PROGRAM MAIN
VAR
	AODB			: ARRAY[0..49] OF ST_IEC870_5_101AODBEntry;(* Application object data base (data points)*)
	hServer			: T_HSERVER;(* Server connection handle *)
	fbServer		: FB_IEC870_5_104SlaveGrp;(* IEC 60870-5-104 controlled station function block instance *)
	aConnections	: ARRAY[0..1] OF ST_IEC870_5_104ServerConnection; (* Two master connections *)

	nCAA			: UDINT := 7;(* Common ASDU address of local (slave) station *)

	inputs AT%I*	: ARRAY[0..2999] OF BYTE;
	outputs AT%Q*	: ARRAY[0..2999] OF BYTE;
	memory AT%M*	: ST_MemoryData;
	data 			: ARRAY[0..2999] OF BYTE;

	bEnable			: BOOL := TRUE;(* Enables/disables communication/data exchange *)
	bBlock			: BOOL;(* Quality flags sample: Rising edge sets BL quality flag to 1 *)
	bUnblock		: BOOL;(* Quality flags sample: Rising edge resets BL quality flag to 0 *)
	bIsBlocked		: BOOL;(* Quality flags sample: BL quality flag status information (TRUE => BL == 1, FALSE => BL == 0) *)
	bSendSpont		: BOOL;(* Sample: TRUE => simulate/modify plc process data (send spontanous data) *)

	fbTimer			: TON := ( PT := T#10S );
	bInit			: BOOL := TRUE;
	nInitErr		: UDINT;
END_VAR

IF bInit THEN
	bInit := FALSE;

	F_CreateServerHnd( '',(* TwinCAT network adress of TCP/IP server, Default = empty string *)
						'127.0.0.1',(* Local (server) address. String containing an (Ipv4) Internet Protocol dotted address. *)
						2404,(* Local (server) Internet Protocol (IP) port. Default = 2404 *)
						nMode := LISTEN_MODE_CLOSEALL OR CONNECT_MODE_ENABLEDBG,(* Close all previous (old) connections and enable debug messages *)
						bEnable, 
						hServer );

	(* Configure protocol parameter *)
	fbServer.protPara.t0				:= T#30S;(* MASTER only: Connection establishment, Default = 30s *)
	fbServer.protPara.t1 				:= T#15S;(* Response Timeout (STARTDTAct, STOPDTAct, TESTFRAct only, Default = 15s ) *)
	fbServer.protPara.t2 				:= T#10S;(* Send ACK in case of no data frames, Default = 10s *)
	fbServer.protPara.t3 				:= T#20S;(* Time for sending test frames, Default = 20s *)
	fbServer.protPara.iK 				:= 12;(* Max. difference RSN to send ACK, Default = 12 *)
	fbServer.protPara.iW 				:= 8;(* Latest ACK after receiving I-frames, Default = 8 *)
	fbServer.protPara.bThrottleMode 	:= TRUE;(* If set reduces the number of polling socket read requests *)
	fbServer.protPara.bPackFrames 		:= TRUE;(* Binds more than one APDU frame to one big TCP/IP frame *)

	(* Configure system parameter *)
	fbServer.sysPara.asduAddr 			:= nCAA;(* Own common ASDU address *)
	fbServer.sysPara.asduFmt.eCOTSize 		:= eIEC870_COT_TwoOctets;(* Cause of transfer octet size *)
	fbServer.sysPara.asduFmt.eAsduAddrSize 	:= eIEC870_AsduAddr_TwoOctets;(* Common ASDU address octet size *)
	fbServer.sysPara.asduFmt.eObjAddrSize 	:= eIEC870_ObjAddr_ThreeOctets;(* Object address octet size *)

	fbServer.sysPara.bUsePCTime 		:= TRUE;(* Initialize substation clock with PC time *)
	fbServer.sysPara.bSyncTime 			:= TRUE;(* Clock synchronisation command enabled *)
	fbServer.sysPara.bSyncPCTime 		:= FALSE;(* Synchronisation of PC time disabled *)
	fbServer.sysPara.bTimeCOT3 			:= FALSE;(* Transmission of C_CS_NA_1 with COT = spontanous disabled *)

	fbServer.sysPara.bEndOfInit 		:= TRUE;(* Send end of initialization *)

	fbServer.sysPara.bPerCyclic			:= FALSE;(* Periodic, cyclic data transfer disabled *)
	fbServer.sysPara.tPerCyclicBase		:= T#5S;(* Periodic, cyclic data transfer base time *)

	fbServer.sysPara.bBackScan			:= FALSE;(* Background scan disabled *)
	fbServer.sysPara.tBackScanCycle		:= T#30S;(* Background scan cycle time *)

	fbServer.sysPara.bPerFRZ			:= TRUE;(* Periodic freeze/reset of integrated totals enabled *)
	fbServer.sysPara.tPerFRZCycle		:= T#15S;(* Perdiodic freeze/reset of integrate totals cycle time *)

	
	fbServer.sysPara.dbgMode 			:= IEC870_DEBUGMODE_DEVSTATE OR IEC870_DEBUGMODE_LINKERROR(* OR IEC870_DEBUGMODE_ASDU OR IEC870_DEBUGMODE_LINKLAYER *); 



	(* Configure your IEC data points here: *)

	(* Monitored Single Points *)
	nInitErr := F_iecInitAOEntry( M_SP_NA_1, 100, IEC870_GRP_INROGEN, 0, MAP_AREA_MEMORY, ADR( memory.eSPI_100_msg ) - ADR( memory ), 0, AODB[0] );
	nInitErr := F_iecInitAOEntry( M_SP_NA_1, 101, IEC870_GRP_INROGEN, 0, MAP_AREA_MEMORY, ADR( memory.eSPI_101_msg ) - ADR( memory ), 0, AODB[1] );
	nInitErr := F_iecInitAOEntry( M_SP_TB_1, 102, IEC870_GRP_INROGEN, 0, MAP_AREA_MEMORY, ADR( memory.eSPI_102_msg ) - ADR( memory ), 0, AODB[2] );
	(* Double Points*)
	nInitErr := F_iecInitAOEntry( M_DP_NA_1, 200, IEC870_GRP_INROGEN, 0, MAP_AREA_MEMORY, ADR( memory.eDPI_200_msg ) - ADR( memory ), 0, AODB[3] );
	nInitErr := F_iecInitAOEntry( M_DP_NA_1, 201, IEC870_GRP_INROGEN, 0, MAP_AREA_MEMORY, ADR( memory.eDPI_201_msg ) - ADR( memory ), 0, AODB[4] );
	nInitErr := F_iecInitAOEntry( M_DP_TB_1, 202, IEC870_GRP_INROGEN, 0, MAP_AREA_MEMORY, ADR( memory.eDPI_202_msg ) - ADR( memory ), 0, AODB[5] );
	(* Regulating step value *)
	nInitErr := F_iecInitAOEntry( M_ST_NA_1, 300, IEC870_GRP_INROGEN, 0, MAP_AREA_MEMORY, ADR( memory.nVTI_300_msg ) - ADR( memory ), 0, AODB[6] );
	nInitErr := F_iecInitAOEntry( M_ST_NA_1, 301, IEC870_GRP_INROGEN, 0, MAP_AREA_MEMORY, ADR( memory.nVTI_301_msg ) - ADR( memory ), 0, AODB[7] );
	nInitErr := F_iecInitAOEntry( M_ST_TB_1, 302, IEC870_GRP_INROGEN, 0, MAP_AREA_MEMORY, ADR( memory.nVTI_302_msg ) - ADR( memory ), 0, AODB[8] );
	(* 32 bit string*)
	nInitErr := F_iecInitAOEntry( M_BO_NA_1, 400, IEC870_GRP_INROGEN, 0, MAP_AREA_MEMORY, ADR( memory.nBSI_400_msg ) - ADR( memory ), 0, AODB[9] );
	nInitErr := F_iecInitAOEntry( M_BO_NA_1, 401, IEC870_GRP_INROGEN, 0, MAP_AREA_MEMORY, ADR( memory.nBSI_401_msg ) - ADR( memory ), 0, AODB[10] );
	nInitErr := F_iecInitAOEntry( M_BO_TB_1, 402, IEC870_GRP_INROGEN, 0, MAP_AREA_MEMORY, ADR( memory.nBSI_402_msg ) - ADR( memory ), 0, AODB[11] );
	(* Measured value, normalized value *)
	nInitErr := F_iecInitAOEntry( M_ME_NA_1, 500, IEC870_GRP_INROGEN, 0, MAP_AREA_MEMORY, ADR( memory.nNVA_500_msg ) - ADR( memory ), 0, AODB[12] );
	nInitErr := F_iecInitAOEntry( M_ME_NA_1, 501, IEC870_GRP_INROGEN, 0, MAP_AREA_MEMORY, ADR( memory.nNVA_501_msg ) - ADR( memory ), 0, AODB[13] );
	nInitErr := F_iecInitAOEntry( M_ME_TD_1, 502, IEC870_GRP_INROGEN, 0, MAP_AREA_MEMORY, ADR( memory.nNVA_502_msg ) - ADR( memory ), 0, AODB[14] );
	(* Mesured value, scaled value *)
	nInitErr := F_iecInitAOEntry( M_ME_NB_1, 600, IEC870_GRP_INROGEN, 0, MAP_AREA_MEMORY, ADR( memory.nSVA_600_msg ) - ADR( memory ), 0, AODB[15] );
	nInitErr := F_iecInitAOEntry( M_ME_NB_1, 601, IEC870_GRP_INROGEN, 0, MAP_AREA_MEMORY, ADR( memory.nSVA_601_msg ) - ADR( memory ), 0, AODB[16] );
	nInitErr := F_iecInitAOEntry( M_ME_TE_1, 602, IEC870_GRP_INROGEN, 0, MAP_AREA_MEMORY, ADR( memory.nSVA_602_msg ) - ADR( memory ), 0, AODB[17] );
	(* Measured value , short floating point value *)
	nInitErr := F_iecInitAOEntry( M_ME_NC_1, 700, IEC870_GRP_INROGEN, 0, MAP_AREA_MEMORY, ADR( memory.fR32_700_msg ) - ADR( memory ), 0, AODB[18] );
	nInitErr := F_iecInitAOEntry( M_ME_NC_1, 701, IEC870_GRP_INROGEN, 0, MAP_AREA_MEMORY, ADR( memory.fR32_701_msg ) - ADR( memory ), 0, AODB[19] );
	nInitErr := F_iecInitAOEntry( M_ME_TF_1, 702, IEC870_GRP_INROGEN, 0, MAP_AREA_MEMORY, ADR( memory.fR32_702_msg ) - ADR( memory ), 0, AODB[20] );

	(* Integrated totals *)
	(* We configure the Mode A: local freeze and spontanous data transfer *)
	nInitErr := F_iecInitAOEntry( M_IT_NA_1, 800, IEC870_GRP_REQCOGEN OR IEC870_GRP_LOCFREEZE, 0, MAP_AREA_MEMORY, ADR( memory.nBCR_800_msg ) - ADR( memory ), 0, AODB[21] );
	nInitErr := F_iecInitAOEntry( M_IT_NA_1, 801, IEC870_GRP_REQCOGEN OR IEC870_GRP_LOCFREEZE, 0, MAP_AREA_MEMORY, ADR( memory.nBCR_801_msg ) - ADR( memory ), 0, AODB[22] );
	nInitErr := F_iecInitAOEntry( M_IT_TB_1, 802, IEC870_GRP_REQCOGEN OR IEC870_GRP_LOCFREEZE, 0, MAP_AREA_MEMORY, ADR( memory.nBCR_802_msg ) - ADR( memory ), 0, AODB[23] );

	(* Controlled Single commands *)
	nInitErr := F_iecInitAOEntry( C_SC_NA_1, 10, 0, 0, MAP_AREA_MEMORY, ADR( memory.eSCS_10_cmd ) - ADR( memory ), 0, AODB[24] );
	nInitErr := F_iecInitAOEntry( C_SC_NA_1, 11, 0, 0, MAP_AREA_MEMORY, ADR( memory.eSCS_11_cmd ) - ADR( memory ), 0, AODB[25] );
	nInitErr := F_iecInitAOEntry( C_SC_TA_1, 12, 0, 0, MAP_AREA_MEMORY, ADR( memory.eSCS_12_cmd ) - ADR( memory ), 0, AODB[26] );
	(* Double commands *)
	nInitErr := F_iecInitAOEntry( C_DC_NA_1, 20, 0, 0, MAP_AREA_MEMORY, ADR( memory.eDCS_20_cmd ) - ADR( memory ), 0, AODB[27] );
	nInitErr := F_iecInitAOEntry( C_DC_NA_1, 21, 0, 0, MAP_AREA_MEMORY, ADR( memory.eDCS_21_cmd ) - ADR( memory ), 0, AODB[28] );
	nInitErr := F_iecInitAOEntry( C_DC_TA_1, 22, 0, 0, MAP_AREA_MEMORY, ADR( memory.eDCS_22_cmd ) - ADR( memory ), 0, AODB[29] );
	(* Regulating step commands *)
	nInitErr := F_iecInitAOEntry( C_RC_NA_1, 30, 0, 0, MAP_AREA_MEMORY, ADR( memory.nVTI_30_cmd ) - ADR( memory ), 0, AODB[30] );
	nInitErr := F_iecInitAOEntry( C_RC_NA_1, 31, 0, 0, MAP_AREA_MEMORY, ADR( memory.nVTI_31_cmd ) - ADR( memory ), 0, AODB[31] );
	nInitErr := F_iecInitAOEntry( C_RC_TA_1, 32, 0, 0, MAP_AREA_MEMORY, ADR( memory.nVTI_32_cmd ) - ADR( memory ), 0, AODB[32] );
	(* 32 bit string commands *)
	nInitErr := F_iecInitAOEntry( C_BO_NA_1, 40, 0, 0, MAP_AREA_MEMORY, ADR( memory.nBSI_40_cmd ) - ADR( memory ), 0, AODB[33] );
	nInitErr := F_iecInitAOEntry( C_BO_NA_1, 41, 0, 0, MAP_AREA_MEMORY, ADR( memory.nBSI_41_cmd ) - ADR( memory ), 0, AODB[34] );
	nInitErr := F_iecInitAOEntry( C_BO_TA_1, 42, 0, 0, MAP_AREA_MEMORY, ADR( memory.nBSI_42_cmd ) - ADR( memory ), 0, AODB[35] );
	(* Set point,  normalized values*)
	nInitErr := F_iecInitAOEntry( C_SE_NA_1, 50, 0, 0, MAP_AREA_MEMORY, ADR( memory.nNVA_50_cmd ) - ADR( memory ), 0, AODB[36] );
	nInitErr := F_iecInitAOEntry( C_SE_NA_1, 51, 0, 0, MAP_AREA_MEMORY, ADR( memory.nNVA_51_cmd ) - ADR( memory ), 0, AODB[37] );
	nInitErr := F_iecInitAOEntry( C_SE_TA_1, 52, 0, 0, MAP_AREA_MEMORY, ADR( memory.nNVA_52_cmd ) - ADR( memory ), 0, AODB[38] );
	(* Set point,  scaled valuess *)
	nInitErr := F_iecInitAOEntry( C_SE_NB_1, 60, 0, 0, MAP_AREA_MEMORY, ADR( memory.nSVA_60_cmd ) - ADR( memory ), 0, AODB[39] );
	nInitErr := F_iecInitAOEntry( C_SE_NB_1, 61, 0, 0, MAP_AREA_MEMORY, ADR( memory.nSVA_61_cmd ) - ADR( memory ), 0, AODB[40] );
	nInitErr := F_iecInitAOEntry( C_SE_TB_1, 62, 0, 0, MAP_AREA_MEMORY, ADR( memory.nSVA_62_cmd ) - ADR( memory ), 0, AODB[41] );
	(* Set point,  short floating point values *)
	nInitErr := F_iecInitAOEntry( C_SE_NC_1, 70, 0, 0, MAP_AREA_MEMORY, ADR( memory.fR32_70_cmd ) - ADR( memory ), 0, AODB[42] );
	nInitErr := F_iecInitAOEntry( C_SE_NC_1, 71, 0, 0, MAP_AREA_MEMORY, ADR( memory.fR32_71_cmd ) - ADR( memory ), 0, AODB[43] );
	nInitErr := F_iecInitAOEntry( C_SE_TC_1, 72, 0, 0, MAP_AREA_MEMORY, ADR( memory.fR32_72_cmd ) - ADR( memory ), 0, AODB[44] );

ELSE
	(* Execute IEC slave function block *)
	fbServer( 	pInputs 		:= ADR( inputs ),
				cbInputs 		:= SIZEOF( inputs ),
				pOutputs 		:= ADR( outputs ),
				cbOutputs 		:= SIZEOF( outputs ),
				pMemory 		:= ADR( memory ),
				cbMemory 		:= SIZEOF( memory ),
				pData 			:= ADR( data ),
				cbData 			:= SIZEOF( data ),
				pAOEntries 		:= ADR( AODB ),
				cbAOEntries 	:= SIZEOF( AODB ),
				pConnections 	:= ADR( aConnections ),
				cbConnections 	:= SIZEOF( aConnections ),
				hServer 		:= hServer,
				bEnable 		:= bEnable );

	(* Check for device errors *)
	REPEAT
		fbServer.system.device.errors.RemoveError();
		IF fbServer.system.device.errors.bOk  THEN
			ADSLOGSTR( 	ADSLOG_MSGTYPE_ERROR OR ADSLOG_MSGTYPE_LOG, 'IEC60870-5-104 slave error: 0x%s',
						DWORD_TO_HEXSTR( fbServer.system.device.errors.getError.nErrId, 8, FALSE) );
		END_IF
	UNTIL NOT fbServer.system.device.errors.bOk
	END_REPEAT

	(* Set block quality flag *)					
	IF bBlock THEN
		bBlock := FALSE;
		F_iecSetAOQuality( IECQ_BL_ON, AODB[0], fbServer.system.device );
	END_IF

	(* Clear block quality flag *)
	IF bUnblock THEN
		bUnblock := FALSE;
		F_iecSetAOQuality( IECQ_BL_OFF, AODB[0], fbServer.system.device );
	END_IF

	(* Check if block quality flag is set *)
	bIsBlocked := SEL( ( F_iecGetAOQuality( AODB[0], fbServer.system.device ) AND IECQ_BL_ON )  = IECQ_BL_ON, FALSE, TRUE );

END_IF

(* Simulate/modify plc process data *)
fbTimer( IN := bSendSpont );
IF fbTimer.Q THEN
	fbTimer( IN := FALSE );
	fbTimer( IN := bSendSpont );

	memory.eSPI_100_msg := SEL( memory.eSPI_100_msg = eIEC870_SPI_OFF, eIEC870_SPI_OFF, eIEC870_SPI_ON );
	memory.eSPI_101_msg := SEL( memory.eSPI_101_msg = eIEC870_SPI_OFF, eIEC870_SPI_OFF, eIEC870_SPI_ON );
	memory.eSPI_102_msg := SEL( memory.eSPI_102_msg = eIEC870_SPI_OFF, eIEC870_SPI_OFF, eIEC870_SPI_ON );

	memory.eDPI_200_msg := SEL( memory.eDPI_200_msg = eIEC870_DPI_OFF, eIEC870_DPI_OFF, eIEC870_DPI_ON );
	memory.eDPI_201_msg := SEL( memory.eDPI_201_msg = eIEC870_DPI_OFF, eIEC870_DPI_OFF, eIEC870_DPI_ON );
	memory.eDPI_202_msg := SEL( memory.eDPI_202_msg = eIEC870_DPI_OFF, eIEC870_DPI_OFF, eIEC870_DPI_ON );
	
	F_iecIncVTI( memory.nVTI_300_msg );
	F_iecDecVTI( memory.nVTI_301_msg );
	F_iecIncVTI( memory.nVTI_302_msg );

	memory.nBSI_400_msg := SEL( memory.nBSI_400_msg = 0, ROL( memory.nBSI_400_msg, 1 ), 16#11111111 );
	memory.nBSI_401_msg := SEL( memory.nBSI_401_msg = 0, ROR( memory.nBSI_401_msg, 1 ), 16#22222222 );
	memory.nBSI_402_msg := SEL( memory.nBSI_402_msg = 0, ROL( memory.nBSI_402_msg, 1 ), 16#33333333 );

	memory.nNVA_500_msg := memory.nNVA_500_msg + 1;
	memory.nNVA_501_msg := memory.nNVA_501_msg - 1;
	memory.nNVA_502_msg := memory.nNVA_502_msg + 2;

	memory.nSVA_600_msg := memory.nSVA_600_msg + 1;
	memory.nSVA_601_msg := memory.nSVA_601_msg - 1;
	memory.nSVA_602_msg := memory.nSVA_602_msg + 2;

	memory.fR32_700_msg	:= memory.fR32_700_msg + 0.1;
	memory.fR32_701_msg	:= memory.fR32_701_msg + 0.2;
	memory.fR32_702_msg	:= memory.fR32_702_msg + 0.3;

	memory.nBCR_800_msg := memory.nBCR_800_msg + 1;
	memory.nBCR_801_msg := memory.nBCR_801_msg + 2;
	memory.nBCR_802_msg := memory.nBCR_802_msg + 3;
END_IF

END_PROGRAM
